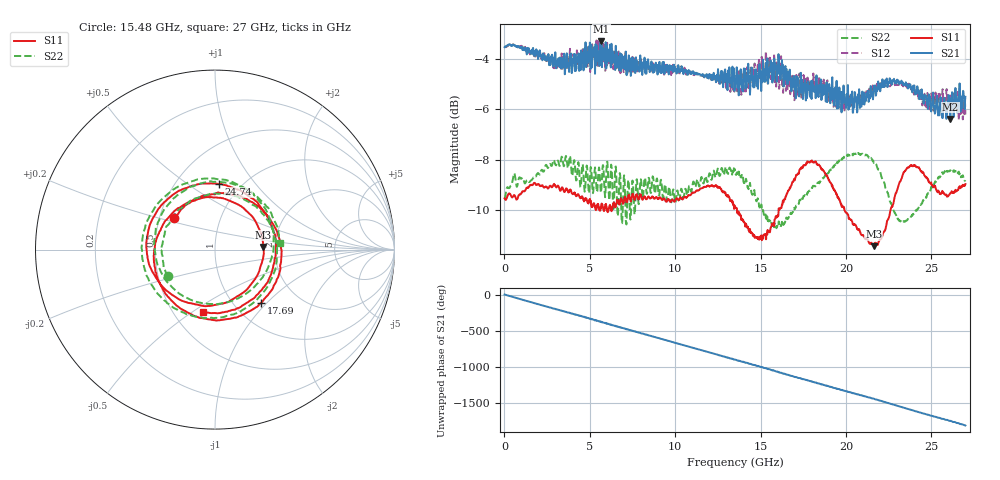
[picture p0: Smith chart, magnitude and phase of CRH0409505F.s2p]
!Agilent Technologies,N5224A,MY51441447,A.10.00.00
!Agilent N5224A: A.10.00.00
!Date: Thursday, November 05, 2015 12:19:24
!Correction: S11(Full 2 Port(1,2))
!S21(Full 2 Port(1,2))
!S12(Full 2 Port(1,2))
!S22(Full 2 Port(1,2))
!S2P File: Measurements: S11, S21, S12, S22:
# Hz S  RI  R 50
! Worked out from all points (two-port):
!   1601 points, 10 MHz to 27 GHz, reference 50 ohm
!   highest |S21| = -3.31 dB at 5.678 GHz (marker M1); lowest = -6.4 dB at 26.12 GHz (marker M2)
!   |S21| within 3 dB of the highest: start of sweep to 25.65 GHz; 26.13 GHz to end of sweep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
!   lowest |S11| = -11.4 dB at 21.64 GHz (marker M3), VSWR 1.73, Z = 86.6 + j2.69 ohm
!   |S11| at or under -10 dB: 6.012 GHz to 6.094 GHz (81.43 MHz wide, 1.35 % of centre); 13.62 GHz to 16.06 GHz (2.439 GHz wide, 16.4 % of centre); 19.93 GHz to 22.61 GHz (2.689 GHz wide, 12.6 % of centre)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
!   |S22| runs from -10.7 to -7.7 dB; largest |S21 - S12| = 0.083
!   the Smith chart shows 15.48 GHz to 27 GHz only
!   S11 on the Smith chart (normalised r, x): 15.48 GHz: 0.60, +0.23; 17.69 GHz: 1.33, -0.93; 24.74 GHz: 0.80, +0.67; 27 GHz: 0.69, -0.56
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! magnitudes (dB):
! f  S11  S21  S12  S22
! 10 MHz  -9.5  -3.5  -3.5  -9.5
! 532.9 MHz  -9.4  -3.5  -3.5  -8.6
! 2.81 GHz  -9.1  -4.0  -4.0  -8.2
! 4.514 GHz  -9.5  -3.9  -3.8  -8.6
! 5.678 GHz  -9.8  -3.3  -4.0  -9.2
! 7.247 GHz  -9.4  -4.4  -4.1  -8.8
! 9.018 GHz  -9.5  -4.3  -4.6  -9.3
! 10.11 GHz  -9.5  -4.4  -4.3  -9.2
! 12.27 GHz  -9.1  -4.6  -4.7  -8.4
! 13.51 GHz  -9.9  -4.9  -4.6  -8.5
! 14.69 GHz  -11.1  -4.4  -4.6  -9.4
! 15.48 GHz  -10.8  -4.5  -4.0  -10.4
! 16.27 GHz  -9.8  -4.3  -4.6  -10.5
! 17.69 GHz  -8.1  -5.1  -4.9  -9.4
! 18.01 GHz  -8.0  -5.1  -4.8  -9.1
! 20.02 GHz  -10.1  -5.8  -5.5  -7.9
! 21.64 GHz  -11.4  -5.1  -5.1  -8.1
! 22.51 GHz  -10.3  -5.0  -5.0  -9.5
! 23.53 GHz  -8.4  -5.0  -5.1  -10.4
! 24.74 GHz  -8.7  -5.8  -5.8  -9.4
! 26.12 GHz  -9.3  -6.4  -5.6  -8.4
! 27 GHz  -9.0  -5.5  -6.2  -8.8
